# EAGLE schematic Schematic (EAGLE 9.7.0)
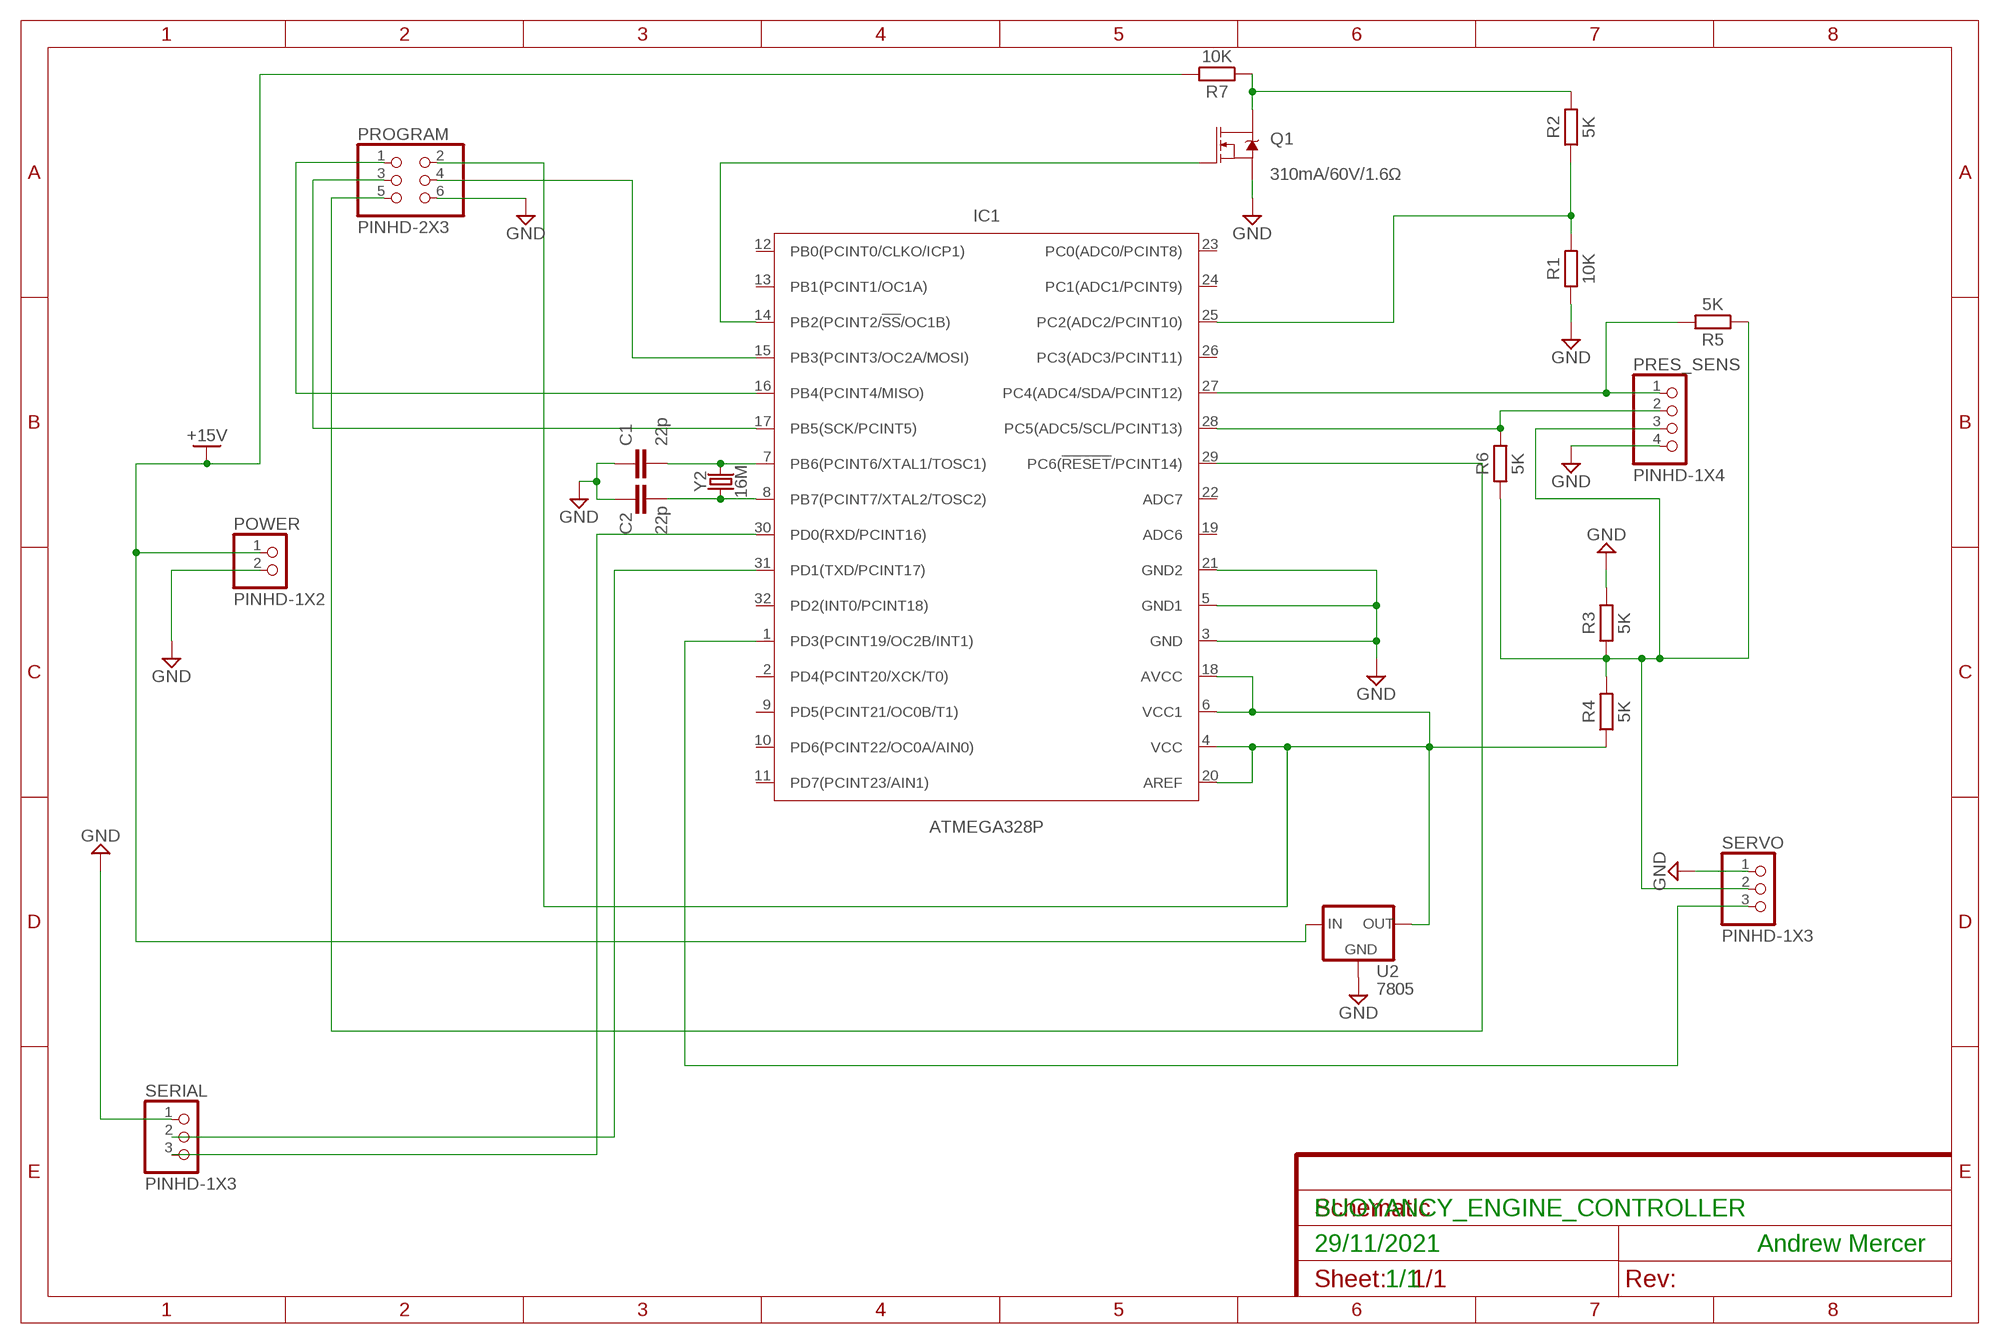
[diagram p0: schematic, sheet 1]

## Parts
C1  22p  C_CHIP-0402(1005-METRIC)  [CAPC1005X60]
C2  22p  C_CHIP-0402(1005-METRIC)  [CAPC1005X60]
IC1  ATMEGA328P  ATMEGA328P_TQFP  [TQFP32-08]
POWER  PINHD-1X2  [1X02]
PRES_SENS  PINHD-1X4  [1X04]
PROGRAM  PINHD-2X3  [2X03]
Q1  310mA/60V/1.6Ω  MOSFET-NCH-2N7002PW  [SOT323]
R1  10K  R_CHIP-0402(1005-METRIC)  [RESC1005X40]
R2  5K  R_CHIP-0402(1005-METRIC)  [RESC1005X40]
R3  5K  R_CHIP-0402(1005-METRIC)  [RESC1005X40]
R4  5K  R_CHIP-0402(1005-METRIC)  [RESC1005X40]
R5  5K  R_CHIP-0402(1005-METRIC)  [RESC1005X40]
R6  5K  R_CHIP-0402(1005-METRIC)  [RESC1005X40]
R7  10K  R_CHIP-0402(1005-METRIC)  [RESC1005X40]
SERIAL  PINHD-1X3  [1X03]
SERVO  PINHD-1X3  [1X03]
U2  7805  V_REG_78XXTO-92_UNTESTED  [TO-92]
Y2  16M  CRYSTALSMD-3.2X1.5  [CRYSTAL-SMD-3.2X1.5MM]

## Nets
+V: POWER.1 R7.2 U2.3(IN) ; supply symbol labelled +15V
GND: C1.1 C2.1 IC1.3(GND) IC1.5(GND1) IC1.21(GND2) POWER.2 PRES_SENS.4 PROGRAM.6 Q1.2(S) R1.1 R3.2 SERIAL.1 SERVO.1 U2.2(GND)
N$1: IC1.4(VCC) IC1.6(VCC1) IC1.18(AVCC) IC1.20(AREF) PROGRAM.2 R4.1 U2.1(OUT)
N$2: C1.2 IC1.7(PB6(PCINT6/XTAL1/TOSC1)) Y2.P$2
N$3: C2.2 IC1.8(PB7(PCINT7/XTAL2/TOSC2)) Y2.P$1
N$4: IC1.28(PC5(ADC5/SCL/PCINT13)) PRES_SENS.2 R6.2
N$5: IC1.27(PC4(ADC4/SDA/PCINT12)) PRES_SENS.1 R5.2
N$7: IC1.14(PB2(PCINT2/!SS!/OC1B)) Q1.1(G)
N$8: IC1.25(PC2(ADC2/PCINT10)) R1.2 R2.1
N$9: Q1.3(D) R2.2 R7.1
N$10: PRES_SENS.3 R3.1 R4.2 R5.1 R6.1 SERVO.2
N$11: IC1.16(PB4(PCINT4/MISO)) PROGRAM.1
N$12: IC1.17(PB5(SCK/PCINT5)) PROGRAM.3
N$13: IC1.29(PC6(!RESET!/PCINT14)) PROGRAM.5
N$14: IC1.15(PB3(PCINT3/OC2A/MOSI)) PROGRAM.4
N$17: IC1.1(PD3(PCINT19/OC2B/INT1)) SERVO.3
N$18: IC1.31(PD1(TXD/PCINT17)) SERIAL.2
N$19: IC1.30(PD0(RXD/PCINT16)) SERIAL.3
Unconnected: IC1.2(PD4(PCINT20/XCK/T0)) IC1.9(PD5(PCINT21/OC0B/T1)) IC1.10(PD6(PCINT22/OC0A/AIN0)) IC1.11(PD7(PCINT23/AIN1)) IC1.12(PB0(PCINT0/CLKO/ICP1)) IC1.13(PB1(PCINT1/OC1A)) IC1.19(ADC6) IC1.22(ADC7) IC1.23(PC0(ADC0/PCINT8)) IC1.24(PC1(ADC1/PCINT9)) IC1.26(PC3(ADC3/PCINT11)) IC1.32(PD2(INT0/PCINT18))

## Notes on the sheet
- BUOYANCY_ENGINE_CONTROLLER
- 29/11/2021 | Andrew Mercer
- 1/1

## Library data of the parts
C1 C2 = Capacitor:C: Capacitor - Generic; CATEGORY: Capacitor
IC1 = IC_Embedded:ATMEGA328P: 8-bit AVR Microcontroller with 32K Bytes In-System Programmable Flash Datasheet; CATEGORY: IC_Embedded; MANUFACTURER: Microchip; MPN: ATmega328P-MMH; OPERATING_TEMP: -40 to 85 °C; PART_STATUS: Active; SUB-CATEGORY: Microcontroller
POWER = Connector:PINHD-1X2: PIN HEADER; CATEGORY: CONNECTOR; SUB-CATEGORY: PIN-HEADER
PRES_SENS = Connector:PINHD-1X4: PIN HEADER; CATEGORY: CONNECTOR; SUB-CATEGORY: PIN-HEADER
PROGRAM = Connector:PINHD-2X3: PIN HEADER; CATEGORY: CONNECTOR; SUB-CATEGORY: PIN-HEADER
Q1 = SparkFun-DiscreteSemi:MOSFET-NCH: N-channel MOSFETs Voltage controlled devices that allow control of high current outputs. SparkFun Products: SparkFun OpenScale SparkFun Digital Sandbox SparkFun Monster Moto Shield SparkFun MOSFET Power Controller; PROD_ID: TRANS-11151
R1-R7 = Resistor:R: Resistor Fixed - Generic; CATEGORY: Resistor; SUB-CATEGORY: Fixed
SERIAL SERVO = Connector:PINHD-1X3: PIN HEADER; CATEGORY: CONNECTOR; SUB-CATEGORY: PIN-HEADER
U2 = SparkFun-IC-Power:V_REG_78XX: Voltage Regulator Standard 78xx regulator. IGO (Input Ground Output). Spark Fun Electronics SKU : COM-00107
Y2 = SparkFun-Clocks:CRYSTAL: Crystals (Generic)

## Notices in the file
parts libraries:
SparkFun-Aesthetics: Licensing: Creative Commons ShareAlike 4.0 International - https://creativecommons.org/licenses/by-sa/4.0
